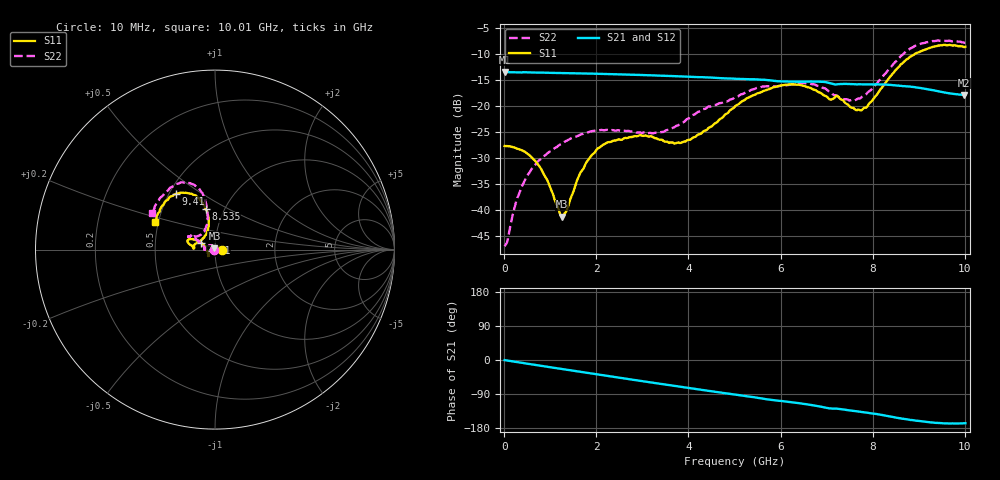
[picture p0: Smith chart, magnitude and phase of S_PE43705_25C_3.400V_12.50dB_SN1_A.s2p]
! Device ID: PE43705
! Serial: 1
! Insertion: A
! Impedance: 50 ohm
! Temp: 25C
! VDD: 3.400V
! Attenuation Step: 12.50dB
#  Hz  S  RI  R  50
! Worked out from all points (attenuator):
!   401 points, 10 MHz to 10.01 GHz, reference 50 ohm
!   highest |S21| = -13.48 dB at 10 MHz (marker M1); lowest = -17.9 dB at 9.985 GHz (marker M2)
!   lowest |S11| = -41.3 dB at 1.26 GHz (marker M3), VSWR 1.02, Z = 49.7 + j0.8 ohm
!   |S11| at or under -10 dB: start of sweep to 8.916 GHz
!   |S22| runs from -46.9 to -7.4 dB; largest |S21 - S12| = 0.0018
!   S11 on the Smith chart (normalised r, x): 10 MHz: 1.09, +0.00; 4.81 GHz: 0.86, +0.06; 8.535 GHz: 0.82, +0.39; 9.41 GHz: 0.54, +0.39; 10.01 GHz: 0.48, +0.17
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1e7  0.0413 0.000132  0.2117 -0.000997  0.2118 -0.000879  -0.00449 0.000419
2.85e8  0.0381 0.00753  0.2093 -0.0204  0.2093 -0.0202  -0.00555 0.0118
4.85e8  0.033 0.0127  0.2073 -0.0344  0.2074 -0.0342  -0.00925 0.0187
8.1e8  0.0189 0.0156  0.2014 -0.0558  0.2014 -0.0557  -0.0198 0.0245
1.26e9  -0.00313 0.00805  0.1894 -0.0837  0.1895 -0.0836  -0.0374 0.0224
1.685e9  -0.0231 -0.00587  0.1746 -0.1079  0.1747 -0.1078  -0.0518 0.0143
2.235e9  -0.0361 -0.0262  0.1511 -0.1353  0.1511 -0.1351  -0.059 0.00181
2.935e9  -0.0389 -0.0349  0.115 -0.1622  0.1152 -0.1621  -0.0558 0.00259
3.36e9  -0.0371 -0.0299  0.0909 -0.1732  0.0911 -0.1731  -0.0548 0.00637
3.985e9  -0.0469 -0.00347  0.0542 -0.1833  0.0543 -0.1831  -0.0713 0.0246
4.81e9  -0.0753 0.0365  0.00676 -0.184  0.0071 -0.184  -0.0979 0.0509
5.01e9  -0.0876 0.0461  -0.00409 -0.1826  -0.00378 -0.1827  -0.1067 0.0576
5.985e9  -0.1461 0.0574  -0.0531 -0.164  -0.0522 -0.1642  -0.136 0.0747
6.685e9  -0.1427 0.0303  -0.0835 -0.1496  -0.0838 -0.1495  -0.1444 0.0721
7.335e9  -0.1101 0.032  -0.1047 -0.1245  -0.1044 -0.1248  -0.0913 0.0775
7.71e9  -0.0657 0.0639  -0.1169 -0.1113  -0.1165 -0.1111  -0.0611 0.1006
8.36e9  -0.0368 0.1837  -0.1363 -0.0832  -0.1355 -0.0838  -0.0438 0.2248
8.535e9  -0.0521 0.225  -0.1391 -0.0724  -0.1383 -0.0739  -0.0549 0.2718
8.935e9  -0.106 0.3016  -0.1417 -0.0515  -0.1412 -0.0511  -0.1183 0.3621
9.41e9  -0.2163 0.3108  -0.1348 -0.0333  -0.1343 -0.0332  -0.2183 0.3647
9.985e9  -0.3282 0.1649  -0.1246 -0.029  -0.1248 -0.0289  -0.3438 0.2137
1.001e10  -0.3354 0.1559  -0.125 -0.0292  -0.1255 -0.0296  -0.3514 0.203
